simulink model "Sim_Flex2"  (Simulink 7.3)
settings: Solver=ode5  StartTime=0.0  StopTime=120  FixedStep=Ts  RelTol=1e-3
InitFcn:
  | r2d= 180/pi; d2r=1/r2d; Ts=0.04;                  % Radian to degree converts
  | [Afls,Bfls,Cfls,Dfls]= vehicle_flex_s;            % Shuttle Ascent, Max_Q, T=55 sec, Flex Vehicle with Slosh and TWD
  | [Aflz,Bflz,Cflz,Dflz]= vehicle_flex_z;            % Discrete Shuttle Plant Model at Max-Q (Flex Vehicle, Actuators, Sensors)
  | [Alfc,Blfc,Clfc,Dlfc]= lateral_fcs;               % Lateral Flight Control System
  | [Apfc,Bpfc,Cpfc,Dpfc]= pitch_fcs;                 % Pitch Flight Control System
  | [Azpl,Bzpl,Czpl,Dzpl]= vehi_plant_z;              % Load Discrete Plant (Vehi,Actuat,Sensors)
  | [Acts,Bcts,Ccts,Dcts]= actuators_5s;              % System of Five Actuators
  | [Actz,Bctz,Cctz,Dctz]= actuators_5z;              % System of Five Actuators, Z-Transform
  | [Asz, Bsz, Csz, Dsz] = sensors_z;                 % IMU, Gyro, Accelerometer Sensors, Z-transform
  | [Aol, Bol, Col, Dol] = open_loop;                 % Open-Loop System (Plant + FCS)
  | load TVC.Mat -ascii                               % Shuttle Stage-1 TVC Matrix at Max-Q
StopFcn:
  | Pl
undefined symbols (not defined in the file or in its folder): Alfc, Apfc, Azpl, Blfc, Bpfc, Bzpl, Clfc, Cpfc, Czpl, Dlfc, Dpfc, Dzpl, TVC

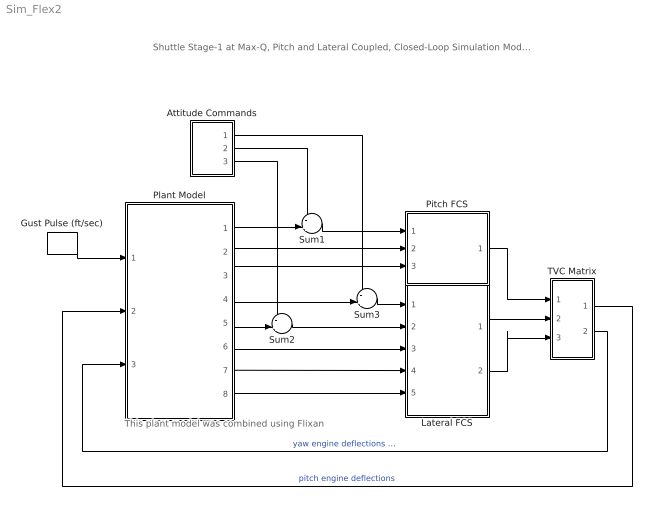
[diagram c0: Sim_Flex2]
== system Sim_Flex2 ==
  note: Shuttle Stage-1 at Max-Q, Pitch and Lateral Coupled, Closed-Loop Simulation Model-2
  note: This plant model was combined using Flixan
  Attitude Commands : Subsystem
  Gust Pulse (ft/sec) : DiscretePulseGenerator  PulseType=Time based  Amplitude=00  Period=200  PulseWidth=2  PhaseDelay=0.12  SampleTime=1
  Lateral FCS : Subsystem
  Pitch FCS : Subsystem
  Plant Model : Subsystem
  Sum1 : Sum  Inputs=-+|  OutDataType=sfix(16)  OutScaling=2^0
  Sum2 : Sum  Inputs=-+|  OutDataType=sfix(16)  OutScaling=2^0
  Sum3 : Sum  Inputs=-+|  OutDataType=sfix(16)  OutScaling=2^0
  TVC Matrix : Subsystem
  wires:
  Plant Model/2(q-flx) -> Pitch FCS/2(q)
  Plant Model/3(Nz) -> Pitch FCS/3(Nz)
  Plant Model/6(p-flx) -> Lateral FCS/3(p)
  Plant Model/7(r-flx) -> Lateral FCS/4(r)
  Plant Model/8(Ny) -> Lateral FCS/5(Ny)
  Sum1/1 -> Pitch FCS/1(theta)
  Plant Model/1(theta) -> Sum1/2
  Gust Pulse (ft/sec)/1 -> Plant Model/1(WG)
  Lateral FCS/1(DP_TVC) -> TVC Matrix/2(roll)
  Pitch FCS/1(DQ_TVC) -> TVC Matrix/1(ptch)
  Lateral FCS/2(DR_TVC) -> TVC Matrix/3(yaw)
  TVC Matrix/2(dz) -> Plant Model/3(dzc)  "yaw engine deflections (rad)"
  TVC Matrix/1(dy) -> Plant Model/2(dyc)  "pitch engine deflections"
  Sum2/1 -> Lateral FCS/2(psi-er)
  Plant Model/5(psi) -> Sum2/2
  Sum3/1 -> Lateral FCS/1(phi-er)
  Plant Model/4(phi) -> Sum3/2
  Attitude Commands/1(roll) -> Sum3/1
  Attitude Commands/2(ptch) -> Sum1/1
  Attitude Commands/3(yaw) -> Sum2/1

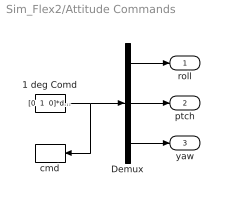
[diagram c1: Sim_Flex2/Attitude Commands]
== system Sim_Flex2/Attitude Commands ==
  1 deg Comd : Constant  Value="[0  1  0]*d2r"  OutDataType=sfix(16)  OutScaling=2^0  SampleTime=-1
  Demux : Demux  Outputs=3
  cmd : ToWorkspace  VariableName=cmd  SampleTime=-1  SaveFormat=Array
  roll : Outport
  ptch : Outport  Port=2
  yaw : Outport  Port=3
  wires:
  Demux/3 -> yaw/1
  Demux/2 -> ptch/1
  Demux/1 -> roll/1
  1 deg Comd/1 -> cmd/1, Demux/1

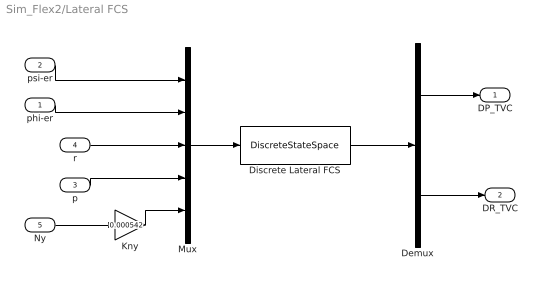
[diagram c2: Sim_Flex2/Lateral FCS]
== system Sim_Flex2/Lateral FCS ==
  phi-er : Inport  OutDataType=sfix(16)  OutScaling=2^0
  psi-er : Inport  Port=2  OutDataType=sfix(16)  OutScaling=2^0
  p : Inport  Port=3  OutDataType=sfix(16)  OutScaling=2^0
  r : Inport  Port=4  OutDataType=sfix(16)  OutScaling=2^0
  Ny : Inport  Port=5  OutDataType=sfix(16)  OutScaling=2^0
  Demux : Demux  Outputs=2
  Discrete Lateral FCS : DiscreteStateSpace  A=Alfc  B=Blfc  C=Clfc  D=Dlfc  SampleTime=Ts
  Kny : Gain  Gain=0.000542  ParameterDataType=sfix(16)  ParameterScaling=2^0  OutDataType=sfix(16)  OutScaling=2^0
  Mux : Mux  Inputs=5
  DP_TVC : Outport  OutDataType=sfix(16)  OutScaling=2^0
  DR_TVC : Outport  Port=2  OutDataType=sfix(16)  OutScaling=2^0
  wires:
  psi-er/1 -> Mux/1
  phi-er/1 -> Mux/2
  r/1 -> Mux/3
  Mux/1 -> Discrete Lateral FCS/1
  Discrete Lateral FCS/1 -> Demux/1
  Demux/1 -> DP_TVC/1
  Demux/2 -> DR_TVC/1
  p/1 -> Mux/4
  Kny/1 -> Mux/5
  Ny/1 -> Kny/1

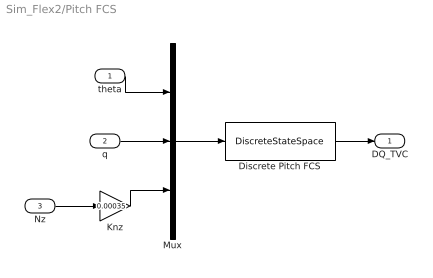
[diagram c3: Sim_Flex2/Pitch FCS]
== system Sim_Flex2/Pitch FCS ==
  theta : Inport  OutDataType=sfix(16)  OutScaling=2^0
  q : Inport  Port=2  OutDataType=sfix(16)  OutScaling=2^0
  Nz : Inport  Port=3  OutDataType=sfix(16)  OutScaling=2^0
  Discrete Pitch FCS : DiscreteStateSpace  A=Apfc  B=Bpfc  C=Cpfc  D=Dpfc  SampleTime=Ts
  Knz : Gain  Gain=0.00035  ParameterDataType=sfix(16)  ParameterScaling=2^0  OutDataType=sfix(16)  OutScaling=2^0
  Mux : Mux  Inputs=3
  DQ_TVC : Outport  OutDataType=sfix(16)  OutScaling=2^0
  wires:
  Mux/1 -> Discrete Pitch FCS/1
  Nz/1 -> Knz/1
  q/1 -> Mux/2
  theta/1 -> Mux/1
  Discrete Pitch FCS/1 -> DQ_TVC/1
  Knz/1 -> Mux/3

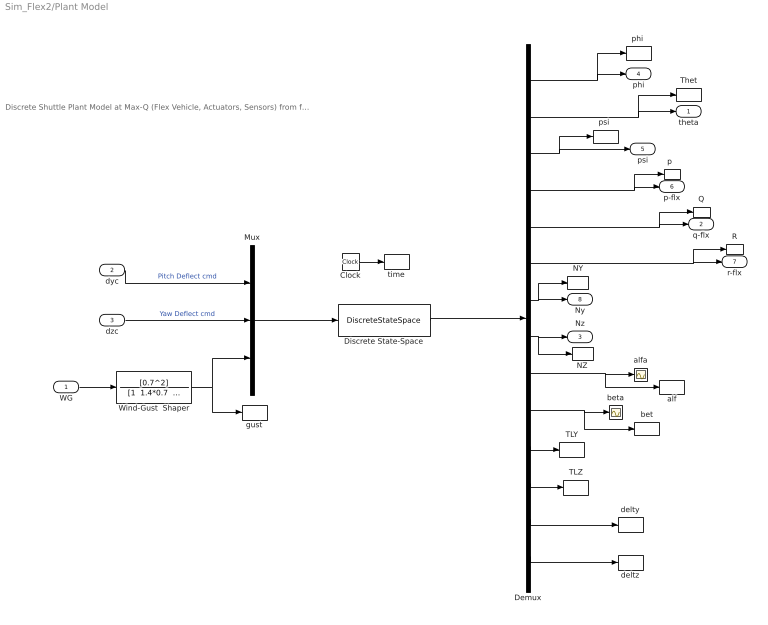
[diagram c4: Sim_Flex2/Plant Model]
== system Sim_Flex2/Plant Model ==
  note: Discrete Shuttle Plant Model at Max-Q (Flex Vehicle, Actuators, Sensors) from file: vehicle_flex_z.m
  WG : Inport  OutDataType=sfix(16)  OutScaling=2^0
  dyc : Inport  Port=2  PortDimensions=5  OutDataType=sfix(16)  OutScaling=2^0
  dzc : Inport  Port=3  PortDimensions=5  OutDataType=sfix(16)  OutScaling=2^0
  Clock : Clock
  Demux : Demux  Outputs=[1,1,1,1,1,1,1,1,1,1, 5,5,5,5]
  Discrete State-Space : DiscreteStateSpace  A=Azpl  B=Bzpl  C=Czpl  D=Dzpl  SampleTime=Ts
  Mux : Mux  Inputs="[5  5  1]"
  NY : ToWorkspace  VariableName=Ny  SampleTime=-1  SaveFormat=Array
  NZ : ToWorkspace  VariableName=Nz  SampleTime=-1  SaveFormat=Array
  Q : ToWorkspace  VariableName=q  SampleTime=-1  SaveFormat=Array
  R : ToWorkspace  VariableName=r  SampleTime=-1  SaveFormat=Array
  TLY : ToWorkspace  VariableName=TLy  SampleTime=-1  SaveFormat=Array
  TLZ : ToWorkspace  VariableName=TLz  SampleTime=-1  SaveFormat=Array
  Thet : ToWorkspace  VariableName=theta  SampleTime=-1  SaveFormat=Array
  Wind-Gust  Shaper : TransferFcn  Numerator=[0.7^2]  Denominator="[1  1.4*0.7  0.7^2]"
  alf : ToWorkspace  VariableName=alpha  SampleTime=-1  SaveFormat=Array
  alfa : Scope
  bet : ToWorkspace  VariableName=beta  SampleTime=-1  SaveFormat=Array
  beta : Scope
  delty : ToWorkspace  VariableName=delty  SampleTime=-1  SaveFormat=Array
  deltz : ToWorkspace  VariableName=deltz  SampleTime=-1  SaveFormat=Array
  gust : ToWorkspace  VariableName=Gust  SampleTime=-1  SaveFormat=Array
  "p  " : ToWorkspace  VariableName=p  SampleTime=-1  SaveFormat=Array
  "phi " : ToWorkspace  VariableName=phi  SampleTime=-1  SaveFormat=Array
  "psi " : ToWorkspace  VariableName=psi  SampleTime=-1  SaveFormat=Array
  time : ToWorkspace  VariableName=time  SampleTime=-1  SaveFormat=Array
  theta : Outport  OutDataType=sfix(16)  OutScaling=2^0
  q-flx : Outport  Port=2  OutDataType=sfix(16)  OutScaling=2^0
  Nz : Outport  Port=3  OutDataType=sfix(16)  OutScaling=2^0
  phi : Outport  Port=4  OutDataType=sfix(16)  OutScaling=2^0
  psi : Outport  Port=5  OutDataType=sfix(16)  OutScaling=2^0
  p-flx : Outport  Port=6  OutDataType=sfix(16)  OutScaling=2^0
  r-flx : Outport  Port=7  OutDataType=sfix(16)  OutScaling=2^0
  Ny : Outport  Port=8  OutDataType=sfix(16)  OutScaling=2^0
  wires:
  dyc/1 -> Mux/1  "Pitch Deflect cmd"
  dzc/1 -> Mux/2  "Yaw Deflect cmd"
  WG/1 -> Wind-Gust  Shaper/1
  Mux/1 -> Discrete State-Space/1
  Discrete State-Space/1 -> Demux/1
  Demux/1 -> phi/1, "phi "/1
  Demux/2 -> theta/1, Thet/1
  Demux/3 -> psi/1, "psi "/1
  Demux/4 -> p-flx/1, "p  "/1
  Demux/5 -> q-flx/1, Q/1
  Demux/6 -> r-flx/1, R/1
  Demux/7 -> Ny/1, NY/1
  Demux/8 -> Nz/1, NZ/1
  Demux/9 -> alfa/1, alf/1
  Demux/10 -> beta/1, bet/1
  Demux/11 -> TLY/1
  Demux/12 -> TLZ/1
  Clock/1 -> time/1
  Demux/13 -> delty/1
  Demux/14 -> deltz/1
  Wind-Gust  Shaper/1 -> Mux/3, gust/1

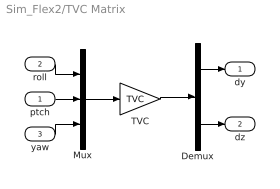
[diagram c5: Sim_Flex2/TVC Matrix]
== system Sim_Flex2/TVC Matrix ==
  ptch : Inport  OutDataType=sfix(16)  OutScaling=2^0
  roll : Inport  Port=2  OutDataType=sfix(16)  OutScaling=2^0
  yaw : Inport  Port=3  OutDataType=sfix(16)  OutScaling=2^0
  Demux : Demux  Outputs="[5  5]"
  Mux : Mux  Inputs=3
  TVC : Gain  Gain=TVC  Multiplication=Matrix(K*u) (u vector)  ParameterDataType=sfix(16)  ParameterScaling=2^0  OutDataType=sfix(16)  OutScaling=2^0
  dy : Outport  OutDataType=sfix(16)  OutScaling=2^0
  dz : Outport  Port=2  OutDataType=sfix(16)  OutScaling=2^0
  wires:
  TVC/1 -> Demux/1
  Mux/1 -> TVC/1
  roll/1 -> Mux/1
  Demux/1 -> dy/1
  ptch/1 -> Mux/2
  Demux/2 -> dz/1
  yaw/1 -> Mux/3
